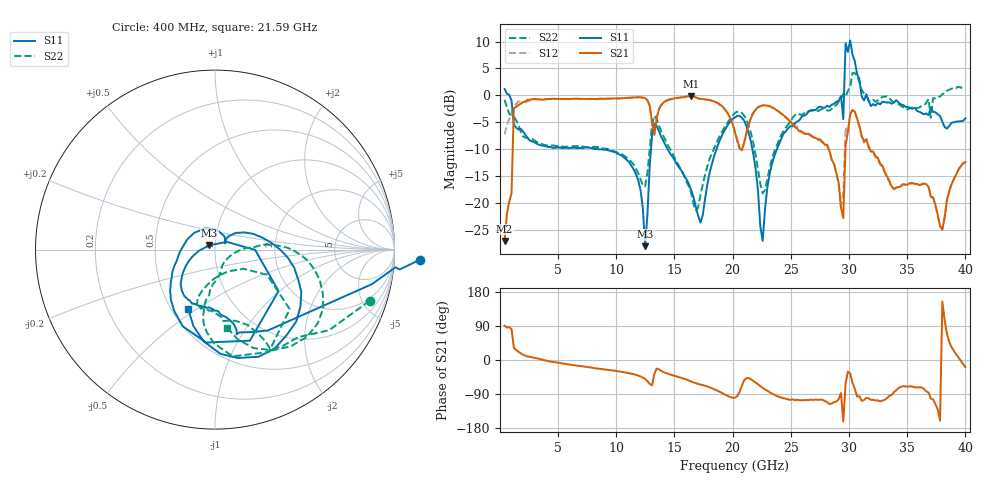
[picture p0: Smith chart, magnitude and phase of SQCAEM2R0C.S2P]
! Network Analyzer HP8722ES.07.66: Jul 25, 2000 Serial No. US39175408
! 26 Oct 2004  11:42:35
! Frequency  S11  S21  S12  S22
# HZ  S  DB R  50
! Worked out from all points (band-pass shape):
!   201 points, 400 MHz to 40 GHz, reference 50 ohm
!   highest |S21| = -0.16 dB at 16.44 GHz (marker M1); lowest = -27.1 dB at 400 MHz (marker M2)
!   |S21| within 3 dB of the highest: 1.183 GHz to 12.95 GHz (11.77 GHz wide, 167 % of centre); 13.6 GHz to 19.51 GHz (5.915 GHz wide, 35.7 % of centre)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
!   lowest |S11| = -28.1 dB at 12.48 GHz (marker M3), VSWR 1.08, Z = 46.9 + j2.29 ohm
!   |S11| at or under -10 dB: 8.384 GHz to 12.98 GHz (4.598 GHz wide, 43 % of centre); 14.4 GHz to 18.61 GHz (4.208 GHz wide, 25.5 % of centre); 21.69 GHz to 23.81 GHz (2.117 GHz wide, 9.3 % of centre)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
!   |S22| runs from -21.4 to 4.2 dB; largest |S21 - S12| = 0.61
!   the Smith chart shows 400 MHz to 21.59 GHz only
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4e8  1.18 -2.8  -27.14 90.5  -7.27 70.9  -0.84 -18.3
1.192e9  -5.38 -56.9  -2.40 32.8  -2.32 28.1  -3.92 -61.0
7.132e9  -9.81 -111.4  -0.67 -16.8  -0.70 -17.5  -9.54 -103.9
1.129e10  -13.08 -143.9  -0.45 -36.2  -0.44 -36.4  -12.39 -107.2
1.2478e10  -28.09 141.8  -0.54 -50.2  -0.54 -51.0  -16.96 -58.9
1.3666e10  -6.68 -112.8  -2.59 -24.9  -2.52 -25.4  -5.65 -90.7
1.6438e10  -17.70 115.2  -0.16 -56.5  -0.15 -57.0  -18.26 -74.8
2.02e10  -4.12 -50.2  -6.85 -99.9  -6.86 -100.0  -3.27 -28.5
2.2576e10  -27.10 -42.3  -1.84 -73.1  -1.89 -73.4  -18.27 -41.7
2.6932e10  -2.72 -43.4  -7.83 -105.3  -7.72 -105.8  -2.83 -4.5
2.8912e10  -1.19 -37.1  -14.49 -109.7  -14.58 -110.3  -1.84 2.3
2.9506e10  -4.44 26.2  -22.88 -162.2  -18.14 -141.9  0.26 27.1
2.9704e10  9.72 -58.9  -9.34 -61.8  -5.94 -49.3  -0.27 -54.1
2.9902e10  8.09 -53.4  -6.75 -30.6  -6.87 -31.0  0.82 8.7
3.01e10  10.22 -68.9  -3.54 -36.0  -3.56 -37.3  1.61 11.9
3.0496e10  6.37 -82.4  -3.07 -76.0  -3.05 -75.2  4.14 -24.3
3.0694e10  3.91 87.1  -4.33 -96.8  -4.42 -96.0  3.59 140.6
3.1288e10  -0.96 91.8  -8.57 -105.7  -8.81 -106.9  0.37 132.0
3.1486e10  0.20 -80.8  -8.15 -99.9  -8.28 -101.5  0.01 -42.8
3.3466e10  -1.33 -66.0  -15.91 -94.6  -16.13 -95.1  -0.45 -32.8
3.6832e10  -3.70 -93.2  -17.01 -86.1  -17.03 -86.5  -0.68 14.0
4e10  -4.26 -70.4  -12.41 -18.8  -12.58 -18.9  1.23 -12.0
